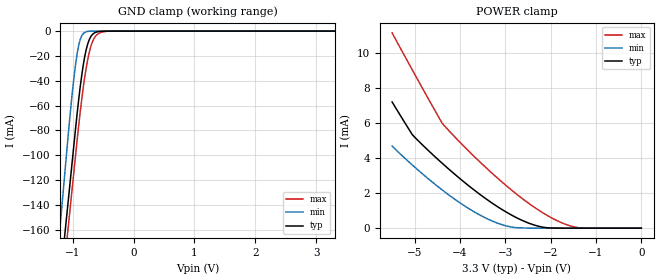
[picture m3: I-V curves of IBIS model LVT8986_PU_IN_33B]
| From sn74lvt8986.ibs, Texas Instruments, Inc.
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[Model]   LVT8986_PU_IN_33B
Model_type  Input
Vinl=0.8
Vinh=2.0
| variable   typ   min   max
C_comp   3.17pF   2.51pF   4.59pF
[Temperature Range]   40   -40   100
| Ambient temperature   25   -40   85
[Voltage range]   3.3   2.7   3.6
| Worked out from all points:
|   GND clamp passes 1 mA (typ) near -0.62 V on its own axis
|   POWER clamp passes 1 mA (typ) near -3.03 V on its own axis
[GND Clamp]
| LVT8986_PU_IN_33B
|   Voltage   I(typ)   I(min)   I(max)
-5.5V     -2.287A    -2.545A    -2.286A
-1.225V   -210.7mA   -168.1mA   -231.2mA
-1.195V   -196.2mA   -151.5mA   -216.8mA
-1.13V    -164.7mA   -115.5mA   -185.6mA
-1.1V     -150.2mA   -98.85mA   -171.2mA
-1.075V   -138.1mA   -85.02mA   -159.2mA
-975mV    -89.72mA   -36.02mA   -111.3mA
-900mV    -54.96mA   -11.41mA   -75.91mA
-775mV    -14.53mA   -496.9uA   -29.08mA
-700mV    -4.283mA   -54.97uA   -12.11mA
-600mV    -648.6uA   -31.02uA   -2.874mA
3.3V      16.16pA    8.699pA    -7.703nA
[POWER Clamp]
| LVT8986_PU_IN_33B
|   Voltage   I(typ)   I(min)   I(max)
-5.5V     7.191mA    4.679mA    11.13mA
-5.055V   5.335mA    3.603mA    9.023mA
-4.39V    3.688mA    2.171mA    5.968mA
-3.895V   2.595mA    1.261mA    4.615mA
-3.45V    1.713mA    598.2uA    3.501mA
-3.055V   1.033mA    183.2uA    2.585mA
-2.715V   547.5uA    22.73uA    1.862mA
-2.17V    55.3uA     4.611nA    869.2uA
-1.83V    1.773uA    15.23pA    391.7uA
-1.525V   8.75nA     13.18pA    99.72uA
-1.26V    93.03pA    11.89pA    5.075uA
-95.1fV   16.16pA    5.854pA    469.5pA
